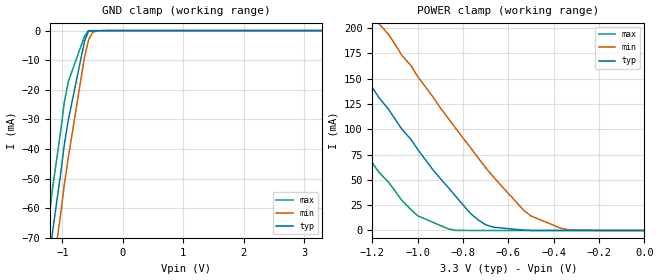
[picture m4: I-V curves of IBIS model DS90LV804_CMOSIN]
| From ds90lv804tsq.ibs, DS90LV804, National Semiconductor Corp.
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[Model]   DS90LV804_CMOSIN
Model_type Input
Vinh=2.0
Vinl=0.8
C_comp   3pF   3pF   3pF
[Model Spec]
S_overshoot_high   3.3   3.0   3.6
S_overshoot_low   0.0   0.0   0.0
[Temperature Range] 25   -40   85
[Voltage Range]   3.3   3.6   3.0
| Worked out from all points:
|   GND clamp passes 1 mA (typ) near -0.58 V on its own axis
|   POWER clamp passes 1 mA (typ) near -0.56 V on its own axis
[GND Clamp]
-3.3V     -416mA     -429mA     -402mA
-1.3V     -89.7mA    -104mA     -74.9mA
-1.23V    -79.3mA    -93mA      -64.5mA
-1.17V    -69.1mA    -82.7mA    -54.4mA
-1.1V     -58.8mA    -72.5mA    -44.3mA
-1.03V    -48.6mA    -62.2mA    -34.2mA
-967mV    -38.4mA    -51.9mA    -24.1mA
-900mV    -30mA      -42.6mA    -17.1mA
-633mV    -3.57mA    -8.92mA    -1.9mA
-567mV    -239uA     -3.14mA    -420nA
-433mV    -133uA     -61.9uA    -233nA
3.3V      21.4pA     6.6nA      19.7pA
[POWER Clamp]
-2.47V    551mA      626mA      475mA
-1.63V    280mA      354mA      203mA
-1.6V     269mA      344mA      193mA
-1.37V    194mA      268mA      118mA
-1.17V    131mA      204mA      57.1mA
-1.13V    120mA      194mA      48mA
-1V       80mA       152mA      14.5mA
-833mV    33.9mA     101mA      60uA
-700mV    5.68mA     61.9mA     6.68uA
-533mV    372uA      20mA       1.71nA
-366mV    1.1uA      2.03mA     12.8pA
0V        6.66pA     6.59nA     6.3pA
